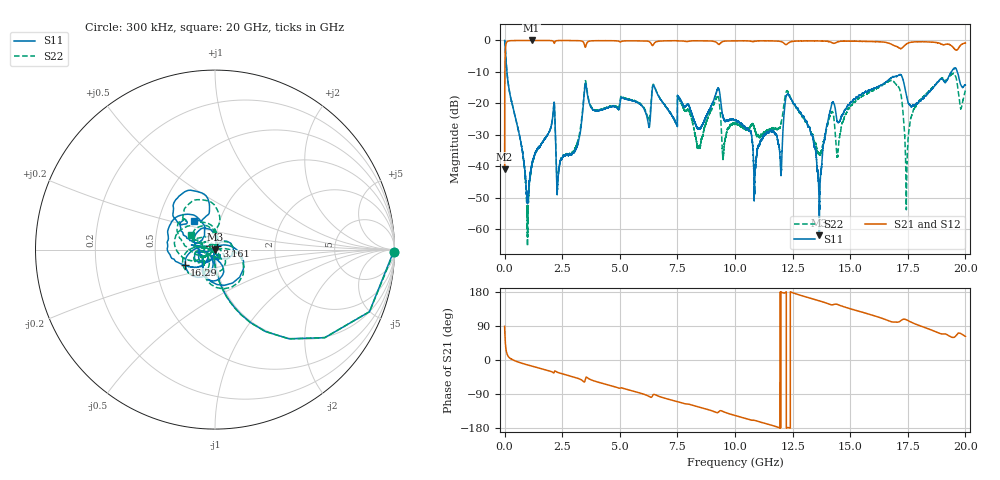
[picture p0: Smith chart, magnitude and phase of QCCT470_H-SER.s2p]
!{QCCT470}
!Johanson Technology Inc.
!www.johansontechnology.com
!Test Board Conditions:
!Substrate Type  RO4350B
!Substrate Thickness  20 mil
!Substrate Dk  3.66
!TL Type: GCPW
!TL Trace Width  34 mil
!TL Gap  10 mil
!Electrode orientation  Horizontal
!DUT TOPOLOGY	SERIES
!Mounting Pad LxW  26x52 mil
! Created Sat Jan  9 19:17:36 2021
# hz S ma R 50
! 2 Port Network Data from SP1.SP block
! freq  magS11  angS11  magS21  angS21  magS12  angS12  magS22  angS22
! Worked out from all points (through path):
!   20001 points, 300 kHz to 20 GHz, reference 50 ohm
!   highest |S21| = 0.00 dB at 1.171 GHz (marker M1); lowest = -41.0 dB at 300 kHz (marker M2)
!   group delay of S21, straight-line fit = 42.4 ps
!   lowest |S11| = -62.0 dB at 13.66 GHz (marker M3), VSWR 1.00, Z = 50.1 - j0.0354 ohm
!   |S11| at or under -10 dB: 99.11 MHz to 19.39 GHz (19.29 GHz wide, 198 % of centre); 19.65 GHz to end of sweep
!   |S22| runs from -65.5 to 0.0 dB; largest |S21 - S12| = 0.014
!   S11 on the Smith chart (normalised r, x): 300 kHz: open; 3.161 GHz: 1.02, +0.04; 16.29 GHz: 0.70, -0.12; 20 GHz: 0.75, +0.25
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300000  0.9948 -0.6  0.008938 88.9  0.009002 89.6  0.9972 -0.8
1.283e8  0.2487 -77.4  0.968 12.6  0.9674 12.6  0.2497 -77.6
9.653e8  0.003141 -153.6  0.9991 -12.4  0.9992 -12.4  0.002015 -79.9
1.1713e9  0.01012 93.8  0.9998 -15.9  0.9984 -15.9  0.009656 59.9
2.0943e9  0.06301 46.8  0.9826 -32.6  0.9829 -32.7  0.06296 44.2
2.3323e9  0.00724 51.3  0.9952 -33.3  0.9957 -33.3  0.007844 36.0
3.1613e9  0.02148 57.2  0.9941 -48.1  0.9928 -48.0  0.02396 9.3
3.3343e9  0.0466 32.8  0.9805 -52.5  0.9809 -52.5  0.05273 6.6
6.6673e9  0.1339 -175.9  0.9705 -95.1  0.9704 -95.1  0.1345 178.1
8.4203e9  0.04025 -125.4  0.9893 -123.9  0.9893 -123.9  0.01988 53.9
1.00003e10  0.05395 -65.4  0.9865 -146.4  0.9888 -146.4  0.04658 -62.2
1.08743e10  0.008476 90.9  0.9726 -159.6  0.9729 -159.7  0.03667 172.1
1.19753e10  0.009514 107.4  0.9645 180.0  0.9647 179.9  0.04386 160.2
1.22903e10  0.1391 129.5  0.8923 -178.2  0.8915 -178.4  0.1545 123.7
1.33343e10  0.03116 75.2  0.9835 161.9  0.985 161.9  0.03181 80.3
1.36613e10  0.0007943 -26.4  0.9817 156.1  0.9825 156.0  0.01522 129.5
1.42143e10  0.1002 -134.3  0.9188 145.5  0.918 145.3  0.07329 155.5
1.62853e10  0.1899 -153.1  0.9527 112.0  0.9466 112.0  0.1846 -165.9
1.66673e10  0.2348 -166.8  0.9099 103.4  0.8984 103.4  0.2236 175.2
1.74503e10  0.1291 116.1  0.8837 105.8  0.885 106.0  0.006226 -149.3
1.81993e10  0.1222 160.7  0.9512 86.7  0.952 86.3  0.1297 -175.1
2e10  0.1967 127.0  0.9088 62.3  0.9023 62.1  0.1598 149.9
